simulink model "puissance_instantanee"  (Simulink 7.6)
settings: Solver=ode23tb  StartTime=0.0  StopTime=0.04  RelTol=1e-3
InitFcn:
  | clc
StopFcn:
  | close all
  | figure (1)
  | load  puiss_instant.mat
  | subplot 211
  | plot(x(1,:),x(4,:),'*',x(1,:),x(5,:))
  | title('Puissances instantanées - Phases A et C')
  | grid
  | xlabel('temps')
  | subplot 212
  | plot(x(1,:),x(2,:),'*',x(1,:),x(3,:))
  | title('Moyenne puissances instantannées')
  | grid
  | xlabel('temps')
  | %%%%%%%%%%%%%%%%%%%%
libraries: powerlib x13, powerlib_extras x4

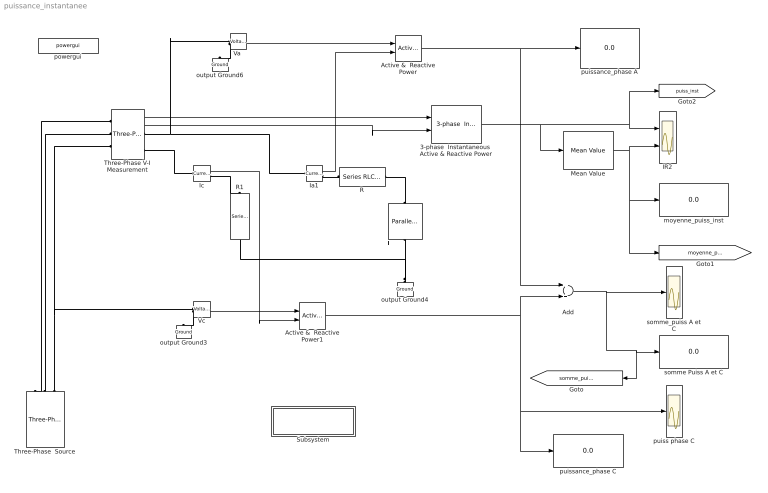
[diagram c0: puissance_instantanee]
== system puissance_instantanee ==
  3-phase  Instantaneous  Active & Reactive Power : powerlib_extras/Measurements/3-phase  Instantaneous  Active & Reactive Power  DialogController=POWERSYS.PowerSysDialog  SystemSampleTime=-1
  Active &  Reactive Power : powerlib_extras/Measurements/Active & Reactive Power  DialogController=POWERSYS.PowerSysDialog  SystemSampleTime=-1  f1=60
  Active &  Reactive Power1 : powerlib_extras/Measurements/Active & Reactive Power  DialogController=POWERSYS.PowerSysDialog  SystemSampleTime=-1  f1=60
  Add : Sum
  IR2 : Scope  NumInputPorts=2
  Ia1 : powerlib/Measurements/Current Measurement  Tag=PoWeRsYsTeMmEaSuReMeNt  DialogController=POWERSYS.PowerSysDialog  SystemSampleTime=-1  PhasorSimulation=off  OutputType=Magnitude  PSBequivalent=0
  Ic : powerlib/Measurements/Current Measurement  Tag=PoWeRsYsTeMmEaSuReMeNt  DialogController=POWERSYS.PowerSysDialog  SystemSampleTime=-1  PhasorSimulation=off  OutputType=Magnitude  PSBequivalent=0
  L : powerlib/Elements/Parallel RLC Branch  DialogController=POWERSYS.PowerSysDialog  PhysicalDomain=powersysdomain  SubClassName=unknown  LeftPortType=p1  RightPortType=p1  LConnTagsString=a  RConnTagsString=__new0  BranchType=L  Resistance=1  Inductance=1e-3  SetiL0=off  InitialCurrent=0  Capacitance=1e-6  Setx0=off  InitialVoltage=0  Measurements=None
  Mean Value : powerlib_extras/Measurements/Mean Value  DialogController=POWERSYS.PowerSysDialog  SystemSampleTime=-1  Period=1/60
  R : powerlib/Elements/Series RLC Branch  DialogController=POWERSYS.PowerSysDialog  PhysicalDomain=powersysdomain  SubClassName=unknown  LeftPortType=p1  RightPortType=p1  LConnTagsString=__new0  RConnTagsString=__new0  BranchType=R  Resistance=1  Inductance=1e-3  SetiL0=off  InitialCurrent=0  Capacitance=1e-6  Setx0=off  InitialVoltage=0  Measurements=None
  R1 : powerlib/Elements/Series RLC Branch  DialogController=POWERSYS.PowerSysDialog  PhysicalDomain=powersysdomain  SubClassName=unknown  LeftPortType=p1  RightPortType=p1  LConnTagsString=__new0  RConnTagsString=__new0  BranchType=R  Resistance=1.8  Inductance=1e-3  SetiL0=off  InitialCurrent=0  Capacitance=1e-6  Setx0=off  InitialVoltage=0  Measurements=None
  Subsystem : Subsystem
  Three-Phase V-I Measurement : powerlib/Measurements/Three-Phase V-I Measurement  DialogController=POWERSYS.PowerSysDialog  SystemSampleTime=-1  VoltageMeasurement=phase-to-ground  SetLabelV=off  LabelV=Vabc  Vpu=off  VpuLL=off  CurrentMeasurement=yes  SetLabelI=off  LabelI=Iabc  Ipu=off  Pbase=100e6  Vbase=500e3  OutputType=Complex  PhasorSimulation=off  PSBequivalent=0
  Three-Phase  Source : powerlib/Electrical Sources/Three-Phase Source  DialogController=POWERSYS.PowerSysDialog  SystemSampleTime=-1  Voltage=220  PhaseAngle=0  Frequency=60  InternalConnection=Yg  SpecifyImpedance=off  Resistance=0  Inductance=0  ShortCircuitLevel=100e6  BaseVoltage=25e3  XRratio=7
  "Va " : powerlib/Measurements/Voltage Measurement  Tag=PoWeRsYsTeMmEaSuReMeNt  DialogController=POWERSYS.PowerSysDialog  SystemSampleTime=-1  PhasorSimulation=off  OutputType=Magnitude  PSBequivalent=0
  Vc : powerlib/Measurements/Voltage Measurement  Tag=PoWeRsYsTeMmEaSuReMeNt  DialogController=POWERSYS.PowerSysDialog  SystemSampleTime=-1  PhasorSimulation=off  OutputType=Magnitude  PSBequivalent=0
  moyenne_puiss_inst : Display
  output Ground3 : powerlib/Elements/Ground  DialogController=POWERSYS.PowerSysDialog  PhysicalDomain=powersysdomain  SubClassName=unknown  LeftPortType=p1  RightPortType=p1  LConnTagsString=a
  output Ground4 : powerlib/Elements/Ground  DialogController=POWERSYS.PowerSysDialog  PhysicalDomain=powersysdomain  SubClassName=unknown  LeftPortType=p1  RightPortType=p1  LConnTagsString=a
  output Ground6 : powerlib/Elements/Ground  DialogController=POWERSYS.PowerSysDialog  PhysicalDomain=powersysdomain  SubClassName=unknown  LeftPortType=p1  RightPortType=p1  LConnTagsString=a
  powergui : powerlib/powergui  Priority=2  SystemSampleTime=-1  SimulationMode=Continuous  SampleTime=0  frequency=60  SPID=off  DisableSnubberDevices=off  DisableRonSwitches=off  DisableVfSwitches=off  SwTol=0  Interpol=off  frequencyindice=60  echomessages=off  HookPort=off  DisplayEquations=off  FunctionMessages=off  EnableUseOfTLC=off  x0status=blocks  RestoreLinks=warning  ResistiveCurrentMeasurement=off  Frange=logspace(0,3,50)  Ylog=off  Xlog=off  ShowGrid=off  save=off  variable=ZData  ZoomFFT=on  StartTime=0.0  cycles=1  DisplayStyle=off  fundamental=60  FreqAxis=off  MaxFrequency=1000  frequencyindicesteady=1  RmsSteady=1  display=off  Ts=0  methode=off
  puiss phase C : Scope
  puissance_phase A : Display
  puissance_phase C : Display
  somme Puiss A et C : Display
  somme_puiss A et C : Scope
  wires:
  "Va "/1 -> Active &  Reactive Power/1
  Active &  Reactive Power/1 -> puissance_phase A/1, Add/1
  Three-Phase V-I Measurement/1 -> 3-phase  Instantaneous  Active & Reactive Power/1
  Three-Phase V-I Measurement/2 -> 3-phase  Instantaneous  Active & Reactive Power/2
  3-phase  Instantaneous  Active & Reactive Power/1 -> Mean Value/1, IR2/1, [puiss_inst]
  Ia1/1 -> Active &  Reactive Power/2
  Ic/1 -> Active &  Reactive Power1/2
  Vc/1 -> Active &  Reactive Power1/1
  Active &  Reactive Power1/1 -> Add/2, puiss phase C/1, puissance_phase C/1
  Add/1 -> somme_puiss A et C/1, somme Puiss A et C/1, [somme_puiss_phases]
  Mean Value/1 -> IR2/2, moyenne_puiss_inst/1, [moyenne_puiss_inst]
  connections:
  Three-Phase V-I Measurement/LConn1 -- Three-Phase  Source/RConn1
  "Va "/LConn2 -- output Ground6/LConn1
  Three-Phase  Source/RConn3 -- Three-Phase V-I Measurement/LConn3 -- Vc/LConn1
  Three-Phase  Source/RConn2 -- Three-Phase V-I Measurement/LConn2
  L/LConn1 -- R/LConn1
  output Ground4/LConn1 -- L/RConn1 -- R1/RConn1
  Ia1/RConn1 -- R/RConn1
  Three-Phase V-I Measurement/RConn1 -- Ia1/LConn1 -- "Va "/LConn1
  Three-Phase V-I Measurement/RConn3 -- Ic/LConn1
  Ic/RConn1 -- R1/LConn1
  Vc/LConn2 -- output Ground3/LConn1

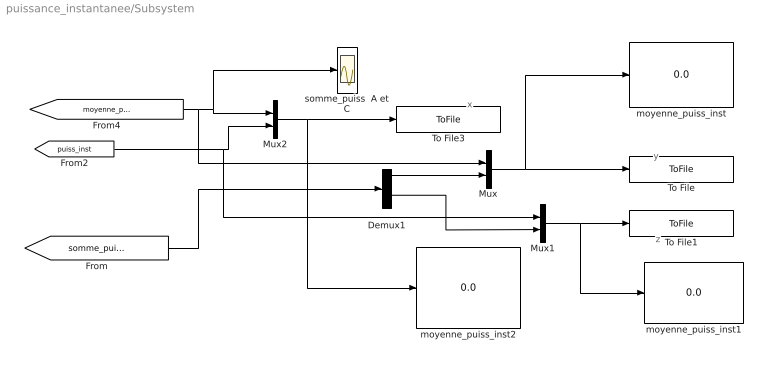
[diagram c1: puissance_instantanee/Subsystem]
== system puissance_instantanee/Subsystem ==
  note: x
  note: y
  note: z
  Demux1 : Demux  Outputs=2
  Mux : Mux  Inputs=2
  Mux1 : Mux  Inputs=2
  Mux2 : Mux  Inputs=2
  To File : ToFile  Filename=puiss_act  MatrixName=y
  To File1 : ToFile  Filename=puiss_react  MatrixName=z
  To File3 : ToFile  Filename=puiss_instant.mat  MatrixName=x
  moyenne_puiss_inst : Display
  moyenne_puiss_inst1 : Display
  moyenne_puiss_inst2 : Display
  somme_puiss  A et C : Scope
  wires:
  [somme_puiss_phases] -> Demux1/1
  Demux1/1 -> Mux/2
  Mux/1 -> To File/1, moyenne_puiss_inst/1
  Demux1/2 -> Mux1/2
  Mux1/1 -> To File1/1, moyenne_puiss_inst1/1
  [puiss_inst] -> Mux2/2, Mux1/1
  [moyenne_puiss_inst] -> Mux2/1, somme_puiss  A et C/1, Mux/1
  Mux2/1 -> To File3/1, moyenne_puiss_inst2/1
